(* Logix 5000 Rung export; software revision 16.04; part 2 of 2 *)
(* AOI56EDNPNET, continued *)

ROUTINE Prescan   (* ladder *)
// Prescan
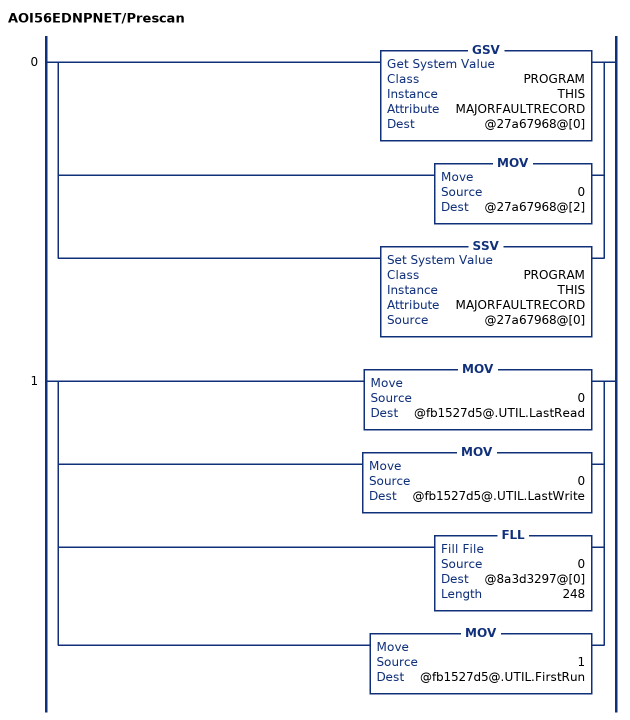
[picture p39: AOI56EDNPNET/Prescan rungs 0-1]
   0: [GSV(PROGRAM,THIS,MAJORFAULTRECORD,@27a67968@[0]) ,MOV(0,@27a67968@[2]) ,SSV(PROGRAM,THIS,MAJORFAULTRECORD,@27a67968@[0]) ];
   1: [MOV(0,@fb1527d5@.UTIL.LastRead) ,MOV(0,@fb1527d5@.UTIL.LastWrite) ,FLL(0,@8a3d3297@[0],248) ,MOV(1,@fb1527d5@.UTIL.FirstRun) ];
END_ROUTINE
END_ADD_ON_INSTRUCTION

VAR_GLOBAL   (* controller tags *)
   AOI56EDNPNET : AOI56EDNPNET;   // Add On Instruction for MVI56-DNPNET Module
   Local:1:O : AB:1756_MODULE_INT_496Bytes:O:0;
   Local:1:I : AB:1756_MODULE_INT_500Bytes:I:0;
   WriteEthernetMSG : MESSAGE;   // Writes IP Addres to the Module
        MessageParameters(MessageType := CIP Generic, RequestedLength := 28, ConnectedFlag := 2, ServiceCode := 16#0010, ObjectType := 16#0004, TargetObject := 8, LocalElement := DNPNET.CONFIG.IP_Settings.IP)
   DNPNET : DNPNETMODULEDEF;
   ReadEthernetMSG : MESSAGE;   // Reads IP Adress from the Module
        MessageParameters(MessageType := CIP Generic, ConnectedFlag := 2, ServiceCode := 16#000e, ObjectType := 16#0004, TargetObject := 8, DestinationTag := DNPNET.CONFIG.IP_Settings.IP)
END_VAR

PROGRAM MainProgram

ROUTINE MainRoutine   (* ladder *)
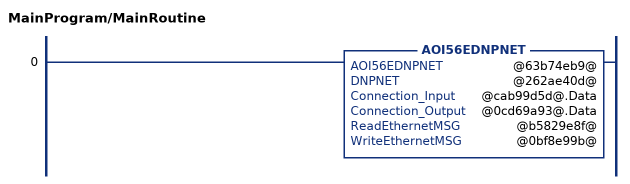
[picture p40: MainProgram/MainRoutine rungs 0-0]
   0: AOI56EDNPNET(@63b74eb9@,@262ae40d@,@cab99d5d@.Data,@0cd69a93@.Data,@b5829e8f@,@0bf8e99b@);
END_ROUTINE
END_PROGRAM
